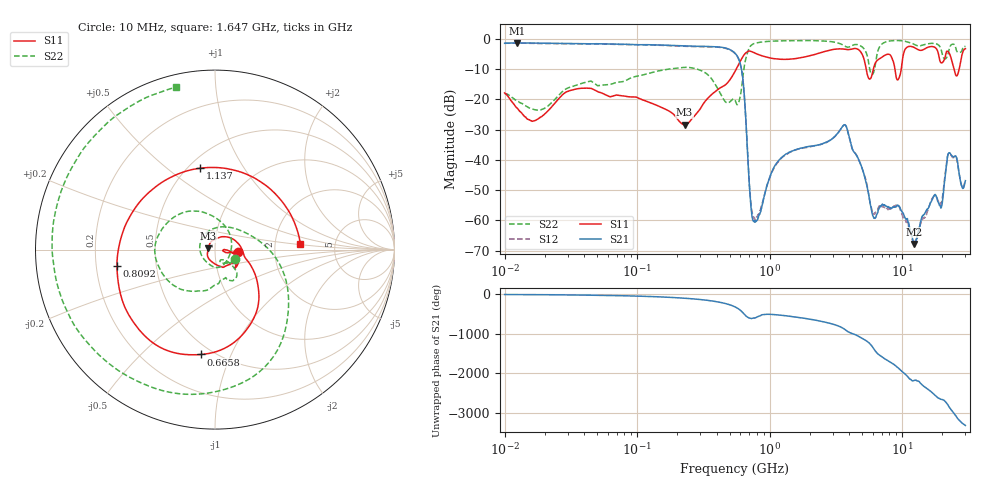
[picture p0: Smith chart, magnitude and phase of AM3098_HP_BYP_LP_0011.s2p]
!Agilent Technologies,E8364B,MY43040894,A.07.50.67
!Agilent E8364B: A.07.50.67
!Date: Wednesday, June 17, 2020 09:19:28
!Correction: S11(Full 2 Port(1,2))
!S21(Full 2 Port(1,2))
!S12(Full 2 Port(1,2))
!S22(Full 2 Port(1,2))
!S2P File: Measurements: S11, S21, S12, S22:Log Frequency Sweep
# Hz S  dB  R 50
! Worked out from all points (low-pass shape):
!   1601 points, 10 MHz to 30 GHz, reference 50 ohm
!   highest |S21| = -1.40 dB at 12.46 MHz (marker M1); lowest = -67.8 dB at 12.25 GHz (marker M2)
!   |S21| within 3 dB of the highest: start of sweep to 535.4 MHz
!   lowest |S11| = -28.4 dB at 228.2 MHz (marker M3), VSWR 1.08, Z = 46.4 + j0.734 ohm
!   |S11| at or under -10 dB: 5.348 GHz to 6.066 GHz (718.1 MHz wide, 12.6 % of centre); 8.813 GHz to 9.845 GHz (1.032 GHz wide, 11.1 % of centre); 24.6 GHz to 26.94 GHz (2.342 GHz wide, 9.09 % of centre)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
!   |S22| runs from -23.6 to -0.6 dB; largest |S21 - S12| = 0.014
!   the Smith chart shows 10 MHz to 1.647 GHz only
!   S11 on the Smith chart (normalised r, x): 10 MHz: 1.29, -0.03; 665.8 MHz: 0.43, -0.78; 809.2 MHz: 0.29, -0.07; 1.137 GHz: 0.57, +0.66; 1.647 GHz: 2.80, +0.24
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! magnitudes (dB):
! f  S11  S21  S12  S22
! 10 MHz  -17.9  -1.5  -1.4  -18.1
! 12.46 MHz  -23.0  -1.4  -1.5  -20.6
! 38.04 MHz  -16.4  -1.7  -1.7  -14.8
! 144.7 MHz  -22.2  -2.1  -2.1  -10.6
! 228.2 MHz  -28.4  -2.4  -2.5  -9.5
! 547.7 MHz  -10.8  -4.8  -4.9  -20.3
! 614.5 MHz  -6.6  -10.4  -10.5  -16.3
! 665.8 MHz  -4.6  -29.0  -29.2  -6.1
! 732.2 MHz  -4.3  -57.9  -56.7  -2.1
! 809.2 MHz  -5.1  -59.8  -58.6  -1.3
! 1.137 GHz  -6.7  -40.9  -41.1  -0.8
! 1.647 GHz  -6.4  -36.4  -36.5  -0.6
! 2.084 GHz  -5.5  -35.5  -35.6  -0.6
! 3.704 GHz  -3.5  -28.4  -28.5  -2.5
! 6.08 GHz  -9.8  -58.9  -57.8  -11.2
! 7.926 GHz  -5.2  -55.7  -56.2  -0.8
! 9.302 GHz  -13.6  -55.0  -54.9  -0.7
! 12.25 GHz  -2.8  -67.8  -67.9  -1.8
! 19.7 GHz  -8.0  -55.8  -54.3  -3.7
! 22.78 GHz  -5.0  -37.6  -37.8  -3.0
! 25.82 GHz  -12.3  -39.5  -39.7  -4.1
! 30 GHz  -3.3  -46.9  -46.7  -2.7
